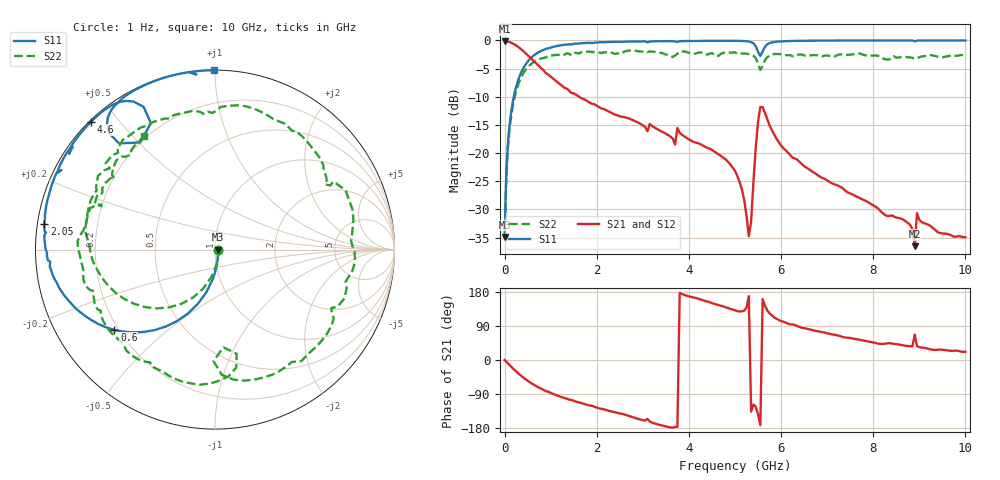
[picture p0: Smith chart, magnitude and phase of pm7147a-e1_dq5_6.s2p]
# GHz S DB R 50
! S-Parameters data
! Freq  dbS11  angS11  dbS21  angS21  dbS12  angS12  dbS22  angS22
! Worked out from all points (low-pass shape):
!   279 points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, 1 Hz to 10 GHz, reference 50 ohm
!   highest |S21| = -0.16 dB at 158.5 Hz (marker M1); lowest = -36.5 dB at 8.9 GHz (marker M2)
!   |S21| within 3 dB of the highest: start of sweep to 570.2 MHz
!   lowest |S11| = -34.9 dB at 158.5 Hz (marker M3), VSWR 1.04, Z = 51.8 - j2.11e-05 ohm
!   |S11| at or under -10 dB: start of sweep to 198.4 MHz
!   |S22| runs from -34.9 to -1.8 dB; largest |S21 - S12| = 0
!   S11 on the Smith chart (normalised r, x): 1 Hz: 1.04, -0.00; 600 MHz: 0.18, -0.34; 2.05 GHz: 0.02, +0.07; 4.6 GHz: 0.00, +0.42; 10 GHz: 0.00, +0.99
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1e-09  -34.91 -0.0  -0.16 0.0  -0.16 0.0  -34.91 -0.0
1.585e-07  -34.91 -0.0  -0.16 -0.0  -0.16 -0.0  -34.91 -0.0
0.05011872  -21.35 -83.1  -0.19 -6.3  -0.19 -6.3  -22.01 -83.9
0.15  -12.23 -101.7  -0.43 -18.6  -0.43 -18.6  -12.93 -106.7
0.6  -2.89 -141.4  -3.40 -62.9  -3.40 -62.9  -4.03 -161.5
0.95  -1.38 -159.0  -6.08 -84.0  -6.08 -84.0  -2.72 171.8
1.7  -0.48 178.7  -10.37 -115.0  -10.37 -115.0  -1.96 130.2
2.05  -0.34 171.5  -11.81 -127.4  -11.81 -127.4  -2.14 111.0
2.75  -0.20 159.3  -14.03 -150.0  -14.03 -150.0  -1.76 77.7
3.35  -0.14 150.6  -15.93 -170.8  -15.93 -170.8  -2.18 43.8
3.95  -0.10 142.7  -17.31 169.6  -17.31 169.6  -2.06 12.2
4.6  -0.07 134.2  -19.99 146.4  -19.99 146.4  -2.79 -26.6
5.05  -0.07 127.9  -24.06 128.8  -24.06 128.8  -2.40 -55.5
5.3  -0.20 122.6  -34.76 168.6  -34.76 168.6  -2.42 -73.0
5.55  -2.76 124.9  -11.81 -172.1  -11.81 -172.1  -5.25 -85.1
5.85  -0.28 126.6  -16.68 112.4  -16.68 112.4  -2.41 -96.4
6.7  -0.04 115.7  -23.38 78.3  -23.38 78.3  -2.59 -142.5
7.65  -0.01 107.1  -27.77 54.7  -27.77 54.7  -2.33 179.3
8.35  -0.01 101.5  -31.16 44.7  -31.16 44.7  -3.38 159.1
8.9  -0.17 96.1  -36.52 66.9  -36.52 66.9  -3.18 143.9
8.95  -0.04 98.0  -30.66 36.6  -30.66 36.6  -3.17 144.7
10  -0.00 90.3  -34.90 21.6  -34.90 21.6  -2.53 122.1
